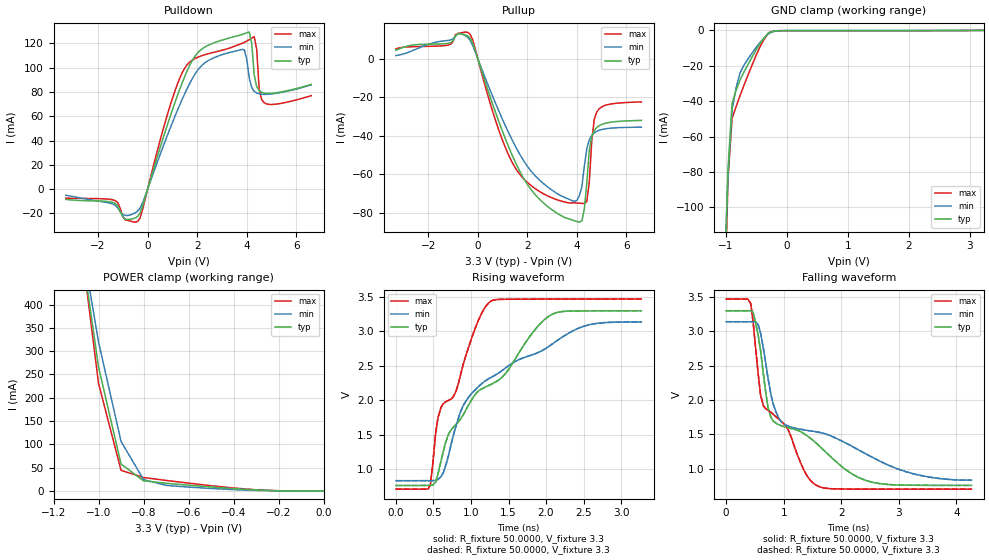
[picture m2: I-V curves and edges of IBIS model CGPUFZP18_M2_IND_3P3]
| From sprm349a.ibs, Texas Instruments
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|   Model Cell CGPUFZP18_M2_IND_3P3
[Model]   CGPUFZP18_M2_IND_3P3
Model_type   I/O
Polarity   Non-Inverting
Enable   Active-Low
Vinl =  0.8
Vinh =  2.0
Cref =  10.0000pF
Rref =  50.0000
Vref =  1.5V
Vmeas =  1.5
C_comp   2.224866p   2.063469p   2.306731p
[Temperature Range]   25   125   -40
[Voltage Range]   3.3   3.14   3.47
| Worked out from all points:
|   slope of the pulldown table from 0 to 0.495 V, typ, clamps not added: 14.8 ohm
|   slope of the pullup table from 0 to 0.495 V, typ, clamps not added: 25.3 ohm
|   GND clamp passes 1 mA (typ) near -0.27 V on its own axis
|   POWER clamp passes 1 mA (typ) near -0.24 V on its own axis
|   rising waveform, R_fixture 50.0000, V_fixture 3.3: 20-80 % time 1.06ns typ, 1.13ns min, 507ps max; typ from 0.761 V to 3.3 V
|   rising waveform, R_fixture 50.0000, V_fixture 3.3: 20-80 % time 1.06ns typ, 1.13ns min, 507ps max; typ from 0.761 V to 3.3 V
|   falling waveform, R_fixture 50.0000, V_fixture 3.3: 20-80 % time 1.11ns typ, 1.59ns min, 719ps max; typ from 3.3 V to 0.758 V
|   falling waveform, R_fixture 50.0000, V_fixture 3.3: 20-80 % time 1.11ns typ, 1.59ns min, 719ps max; typ from 3.3 V to 0.758 V
[POWER_clamp]
|   voltage   I(typ)   I(min)   I(max)
-3.3V     9.989A     8.515A     11.31A
-1.067V   492mA      510.8mA    488.4mA
-1.033V   379.1mA    415.3mA    359.7mA
-1V       266.3mA    319.8mA    231.1mA
-900mV    57.75mA    106.5mA    44.28mA
-800mV    21.77mA    24.36mA    28.75mA
-700mV    16.49mA    11.91mA    22.6mA
-600mV    12.36mA    8.225mA    16.75mA
-300mV    1.972mA    957.1uA    2.414mA
-200mV    320.7uA    154.6uA    343.4uA
-11.55fV  2.899uA    3.969uA    5.984uA
[Pulldown]
|   voltage   I(typ)   I(min)   I(max)
-3.3V     -8.447mA   -5.043mA   -7.456mA
-1.4V     -10.95mA   -12.3mA    -8.83mA
-400mV    -22.4mA    -18.01mA   -26.63mA
1.3V      82.43mA    69.53mA    91.51mA
2.5V      119mA      106.4mA    111.7mA
3.9V      128mA      114.7mA    120.8mA
4.1V      129.3mA    91.31mA    123mA
4.3V      93.96mA    80.57mA    125.6mA
4.4V      84.37mA    79.15mA    115mA
4.5V      81.1mA     78.45mA    82.37mA
4.7V      79.1mA     78.02mA    71.14mA
6.6V      86.19mA    85.82mA    76.95mA
[Pullup]
|   voltage   I(typ)   I(min)   I(max)
-3.3V     4.286mA    1.496mA    4.989mA
-300mV    10.41mA    9.296mA    12.42mA
800mV     -30.78mA   -25.65mA   -35.19mA
1.5V      -53.19mA   -44.94mA   -56.28mA
2.5V      -72.91mA   -62.97mA   -68.85mA
4V        -84.34mA   -73.44mA   -74.76mA
4.2V      -83.95mA   -66.46mA   -74.95mA
4.4V      -64.26mA   -46.53mA   -73.94mA
4.5V      -47.49mA   -42.04mA   -63.86mA
4.7V      -37.3mA    -38.48mA   -31.51mA
5.1V      -33.66mA   -36.49mA   -24.42mA
6.6V      -32.01mA   -35.52mA   -22.44mA
[GND_clamp]
|   voltage   I(typ)   I(min)   I(max)
-3.3V     -13.5A     -11.41A    -15.22A
-1.033V   -153.2mA   -141.9mA   -175.5mA
-966.7mV  -78.78mA   -82.87mA   -84.16mA
-900mV    -41.35mA   -45.23mA   -49.94mA
-833.3mV  -33.83mA   -32.44mA   -43.08mA
-766.7mV  -27.8mA    -23.84mA   -36.66mA
-700mV    -23.24mA   -19.43mA   -30.68mA
-500mV    -10.75mA   -9.357mA   -13.71mA
-366.7mV  -3.998mA   -4.008mA   -4.646mA
-300mV    -1.401mA   -1.842mA   -1.298mA
-100mV    -147.8uA   -94.95uA   -239.5uA
3.233V    -6.106uA   29.44uA    -39.64uA
[Ramp]
| variable   typ   min   max
dV/dt_f   1.52586/1.113433n   1.39287/1.618342n   1.660408/0.7203397n
dV/dt_r   1.295228/1.217725n   1.16499/1.392562n   1.412605/0.6638121n
R_load = 50
[Rising Waveform]
R_fixture = 50.0000
V_fixture = 3.3
V_fixture_min = 3.14
V_fixture_max = 3.47
|   time   V(typ)   V(min)   V(max)
0s        761.4mV    830.9mV    708.1mV
460ps     763mV      831.7mV    776mV
530ps     811.5mV    835.8mV    1.528V
600ps     1.116V     890.8mV    1.894V
760ps     1.602V     1.471V     2.041V
900ps     1.794V     1.928V     2.534V
1.24ns    2.217V     2.316V     3.419V
2.08ns    3.247V     2.814V     3.469V
2.55ns    3.298V     3.089V     3.47V
3.27ns    3.299V     3.137V     3.47V
[Rising Waveform]
R_fixture = 50.0000
V_fixture = 3.3
V_fixture_min = 3.14
V_fixture_max = 3.47
|   time   V(typ)   V(min)   V(max)
0s        761.4mV    830.9mV    708.1mV
460ps     763mV      831.7mV    776mV
530ps     811.5mV    835.8mV    1.528V
600ps     1.116V     890.8mV    1.894V
760ps     1.602V     1.471V     2.041V
900ps     1.794V     1.928V     2.534V
1.24ns    2.217V     2.316V     3.419V
2.08ns    3.247V     2.814V     3.469V
2.55ns    3.298V     3.089V     3.47V
3.27ns    3.299V     3.137V     3.47V
[Falling Waveform]
R_fixture = 50.0000
V_fixture = 3.3
V_fixture_min = 3.14
V_fixture_max = 3.47
|   time   V(typ)   V(min)   V(max)
0s        3.3V       3.14V      3.47V
430ps     3.3V       3.14V      3.401V
560ps     2.929V     3.093V     2.364V
650ps     2.365V     2.742V     1.914V
730ps     1.885V     2.309V     1.847V
910ps     1.642V     1.747V     1.725V
1.52ns    1.406V     1.544V     785.5mV
2.48ns    816.7mV    1.193V     703.2mV
3.32ns    759.4mV    912.8mV    702.7mV
4.26ns    757.5mV    834.5mV    702.7mV
[Falling Waveform]
R_fixture = 50.0000
V_fixture = 3.3
V_fixture_min = 3.14
V_fixture_max = 3.47
|   time   V(typ)   V(min)   V(max)
0s        3.3V       3.14V      3.47V
430ps     3.3V       3.14V      3.401V
560ps     2.929V     3.093V     2.364V
650ps     2.365V     2.742V     1.914V
730ps     1.885V     2.309V     1.847V
910ps     1.642V     1.747V     1.725V
1.52ns    1.406V     1.544V     785.5mV
2.48ns    816.7mV    1.193V     703.2mV
3.32ns    759.4mV    912.8mV    702.7mV
4.26ns    757.5mV    834.5mV    702.7mV
